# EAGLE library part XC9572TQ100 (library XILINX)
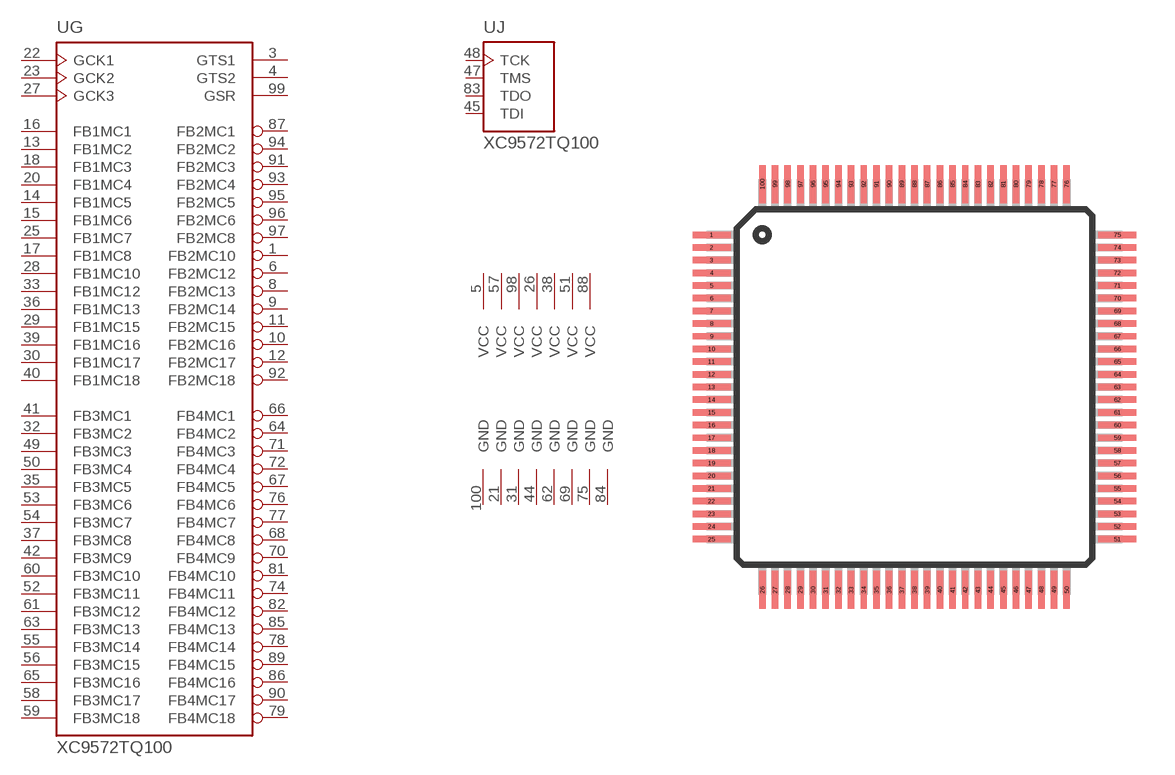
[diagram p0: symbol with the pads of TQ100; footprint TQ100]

Designator prefix -; gates G=XC9572 J=JTAG P=PWR9572TQ100

## XC9572TQ100  [TQ100]
1  G:FB2MC10
3  G:GTS1  in
4  G:GTS2  in
5  P:VCC  pwr
6  G:FB2MC12
8  G:FB2MC13
9  G:FB2MC14
10  G:FB2MC16
11  G:FB2MC15
12  G:FB2MC17
13  G:FB1MC2
14  G:FB1MC5
15  G:FB1MC6
16  G:FB1MC1
17  G:FB1MC8
18  G:FB1MC3
20  G:FB1MC4
21  P:GND  pwr
22  G:GCK1  in
23  G:GCK2  in
25  G:FB1MC7
26  P:VCC  pwr
27  G:GCK3  in
28  G:FB1MC10
29  G:FB1MC15
30  G:FB1MC17
31  P:GND  pwr
32  G:FB3MC2
33  G:FB1MC12
35  G:FB3MC5
36  G:FB1MC13
37  G:FB3MC8
38  P:VCC  pwr
39  G:FB1MC16
40  G:FB1MC18
41  G:FB3MC1
42  G:FB3MC9
44  P:GND  pwr
45  J:TDI  in
47  J:TMS  in
48  J:TCK  in
49  G:FB3MC3
50  G:FB3MC4
51  P:VCC  pwr
52  G:FB3MC11
53  G:FB3MC6
54  G:FB3MC7
55  G:FB3MC14
56  G:FB3MC15
57  P:VCC  pwr
58  G:FB3MC17
59  G:FB3MC18
60  G:FB3MC10
61  G:FB3MC12
62  P:GND  pwr
63  G:FB3MC13
64  G:FB4MC2
65  G:FB3MC16
66  G:FB4MC1
67  G:FB4MC5
68  G:FB4MC8
69  P:GND  pwr
70  G:FB4MC9
71  G:FB4MC3
72  G:FB4MC4
74  G:FB4MC11
75  P:GND  pwr
76  G:FB4MC6
77  G:FB4MC7
78  G:FB4MC14
79  G:FB4MC18
81  G:FB4MC10
82  G:FB4MC12
83  J:TDO  out
84  P:GND  pwr
85  G:FB4MC13
86  G:FB4MC16
87  G:FB2MC1
88  P:VCC  pwr
89  G:FB4MC15
90  G:FB4MC17
91  G:FB2MC3
92  G:FB2MC18
93  G:FB2MC4
94  G:FB2MC2
95  G:FB2MC5
96  G:FB2MC6
97  G:FB2MC8
98  P:VCC  pwr
99  G:GSR  in
100  P:GND  pwr

## Footprint TQ100 (pad centres in mm)
smd 1.5 x 0.254: 1 -8,6; 2 -8,5.5; 3 -8,5; 4 -8,4.5; 5 -8,4; 6 -8,3.5; 7 -8,3; 8 -8,2.5; 9 -8,2; 10 -8,1.5; 11 -8,1; 12 -8,0.5; 13 -8,0; 14 -8,-0.5; 15 -8,-1; 16 -8,-1.5; 17 -8,-2; 18 -8,-2.5; 19 -8,-3; 20 -8,-3.5; 21 -8,-4; 22 -8,-4.5; 23 -8,-5; 24 -8,-5.5; 25 -8,-6; 51 8,-6; 52 8,-5.5; 53 8,-5; 54 8,-4.5; 55 8,-4; 56 8,-3.5; 57 8,-3; 58 8,-2.5; 59 8,-2; 60 8,-1.5; 61 8,-1; 62 8,-0.5; 63 8,0; 64 8,0.5; 65 8,1; 66 8,1.5; 67 8,2; 68 8,2.5; 69 8,3; 70 8,3.5; 71 8,4; 72 8,4.5; 73 8,5; 74 8,5.5; 75 8,6
smd 0.254 x 1.5: 26 -6,-8; 27 -5.5,-8; 28 -5,-8; 29 -4.5,-8; 30 -4,-8; 31 -3.5,-8; 32 -3,-8; 33 -2.5,-8; 34 -2,-8; 35 -1.5,-8; 36 -1,-8; 37 -0.5,-8; 38 0,-8; 39 0.5,-8; 40 1,-8; 41 1.5,-8; 42 2,-8; 43 2.5,-8; 44 3,-8; 45 3.5,-8; 46 4,-8; 47 4.5,-8; 48 5,-8; 49 5.5,-8; 50 6,-8; 76 6,8; 77 5.5,8; 78 5,8; 79 4.5,8; 80 4,8; 81 3.5,8; 82 3,8; 83 2.5,8; 84 2,8; 85 1.5,8; 86 1,8; 87 0.5,8; 88 0,8; 89 -0.5,8; 90 -1,8; 91 -1.5,8; 92 -2,8; 93 -2.5,8; 94 -3,8; 95 -3.5,8; 96 -4,8; 97 -4.5,8; 98 -5,8; 99 -5.5,8; 100 -6,8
